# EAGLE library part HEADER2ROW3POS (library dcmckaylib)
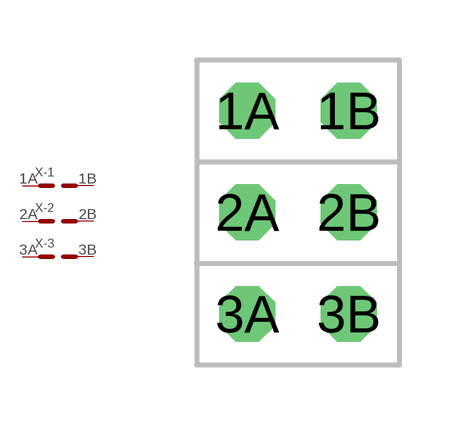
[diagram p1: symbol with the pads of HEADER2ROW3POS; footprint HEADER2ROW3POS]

Designator prefix X; gates -1=HEADER2ROW -2=HEADER2ROW -3=HEADER2ROW

## HEADER2ROW3POS  [HEADER2ROW3POS]
1A  -1:P$1
1B  -1:P$2
2A  -2:P$1
2B  -2:P$2
3A  -3:P$1
3B  -3:P$2

## Footprint HEADER2ROW3POS (pad centres in mm)
drill 0.889 octagon: 1A -1.27,1.27; 1B 1.27,1.27; 2A -1.27,-1.27; 2B 1.27,-1.27; 3A -1.27,-3.81; 3B 1.27,-3.81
